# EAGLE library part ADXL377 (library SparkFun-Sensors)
Analog Devices ADXL377 Low Power 3-Axis ±200 g Accelerometer with Analog Output The ADXL377 is a small, thin, low power, complete 3-axis accelerometer with signal conditioned voltage outputs. The ADXL377 measures acceleration resulting from motion, shock, or vibration with a typical full-scale range of ±200g. Datasheet SparkFun Products SparkFun Triple Axis Accelerometer Breakout - ADXL377 (SEN-12803)
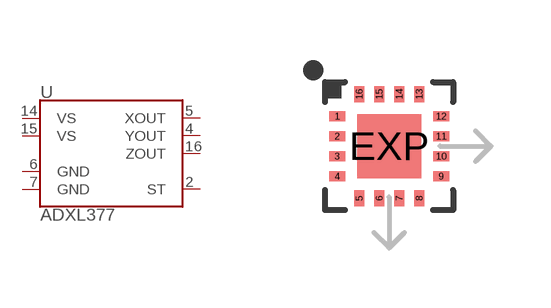
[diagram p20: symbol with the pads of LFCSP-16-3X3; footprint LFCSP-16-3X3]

Designator prefix U

## ADXL377 (PROD_ID: IC-12027)  [LFCSP-16-3X3]
2  ST
4  YOUT
5  XOUT
6  GND
7  GND
14  VS
15  VS
16  ZOUT

## Footprint LFCSP-16-3X3 (pad centres in mm)
16-Pin Lead Frame Chip Scale (LFCSP) w/ Center Pad (3 x 3 mm) Datasheet Specifications: Pin Count: 16 (+ center pad) Area: 3.0 x 3.0 x 1.45 mm Pitch: 0.5 mm Devices Using: ADXL337 ADXL377
smd 0.4 x 0.25: 1 -1.3,0.75; 2 -1.3,0.25; 3 -1.3,-0.25; 4 -1.3,-0.75; 9 1.3,-0.75; 10 1.3,-0.25; 11 1.3,0.25; 12 1.3,0.75
smd 0.25 x 0.4: 5 -0.75,-1.3; 6 -0.25,-1.3; 7 0.25,-1.3; 8 0.75,-1.3; 13 0.75,1.3; 14 0.25,1.3; 15 -0.25,1.3; 16 -0.75,1.3
smd 1.6 x 1.6: EXP 0,0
